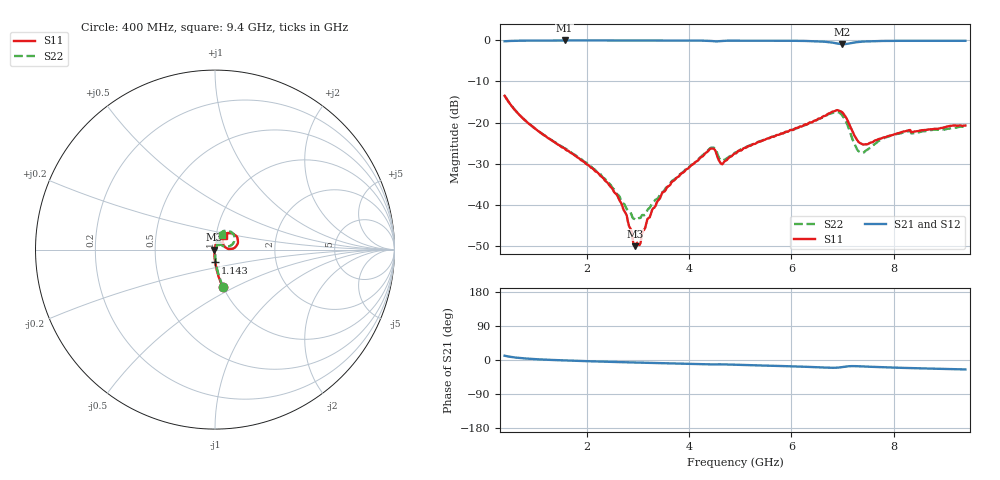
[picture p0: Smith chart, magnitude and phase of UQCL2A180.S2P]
! AVX Corporation
! Date:  10/27/06
! Part No:  UQCL2A180
! Description:  Ultra Low ESR Microwave capacitors
! Mounting Orientation:  Horizontal
# GHZ S DB R 50
! Freq  |S11|  S11 Ph  |S21|  S21 Ph  |S12|  S12 Ph  |S22|  S22 Ph
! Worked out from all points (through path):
!   401 points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, 400 MHz to 9.4 GHz, reference 50 ohm
!   highest |S21| = -0.01 dB at 1.57 GHz (marker M1); lowest = -0.9 dB at 6.993 GHz (marker M2)
!   group delay of S21, straight-line fit = 8.8 ps
!   lowest |S11| = -50.1 dB at 2.943 GHz (marker M3), VSWR 1.01, Z = 49.7 - j0.115 ohm
!   |S11| at or under -10 dB: start of sweep to end of sweep
!   |S22| runs from -43.7 to -13.4 dB; largest |S21 - S12| = 0.0089
!   S11 on the Smith chart (normalised r, x): 400 MHz: 1.00, -0.43; 1.143 GHz: 0.99, -0.14; 9.4 GHz: 1.09, +0.17
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0.4  -13.49 -78.3  -0.21 11.2  -0.20 11.2  -13.45 -77.7
1.143  -22.89 -88.9  -0.03 1.2  -0.02 1.2  -22.81 -86.3
1.57  -26.30 -92.2  -0.01 -1.1  0.00 -1.2  -26.27 -87.1
1.908  -29.30 -94.2  -0.01 -2.7  0.00 -2.7  -29.02 -86.4
2.583  -37.45 -103.0  -0.02 -5.3  0.00 -5.4  -37.32 -74.8
2.74  -41.62 -112.1  -0.02 -5.9  0.00 -5.9  -39.88 -61.1
2.943  -50.12 -158.2  -0.01 -6.6  0.00 -6.7  -43.51 -25.4
3.033  -49.86 146.6  -0.02 -6.9  0.00 -7.0  -43.25 -3.9
3.235  -43.09 101.7  -0.02 -7.7  -0.01 -7.7  -40.76 31.0
3.415  -38.76 93.7  -0.02 -8.2  -0.01 -8.3  -38.03 48.4
3.708  -34.15 85.4  -0.02 -9.3  -0.02 -9.4  -33.92 61.0
4.405  -26.54 65.8  -0.11 -12.0  -0.11 -12.1  -26.35 62.2
4.495  -26.47 51.4  -0.21 -12.0  -0.21 -12.1  -26.19 50.3
4.653  -30.15 59.1  -0.13 -11.5  -0.13 -11.6  -29.20 55.5
4.9  -27.54 69.4  -0.05 -12.6  -0.06 -12.6  -27.35 70.3
6.408  -19.94 57.6  -0.17 -18.6  -0.16 -18.1  -19.95 70.2
6.835  -17.27 37.1  -0.61 -20.6  -0.55 -20.4  -17.54 48.7
6.993  -17.48 17.0  -0.91 -18.7  -0.86 -18.8  -18.24 27.4
7.24  -23.39 6.1  -0.50 -16.2  -0.47 -16.3  -25.37 19.0
7.353  -25.05 19.1  -0.33 -16.7  -0.31 -16.8  -27.23 40.3
7.915  -23.22 50.6  -0.11 -19.7  -0.11 -19.7  -23.36 72.6
9.4  -20.73 56.2  -0.10 -24.9  -0.09 -24.8  -20.90 64.0
